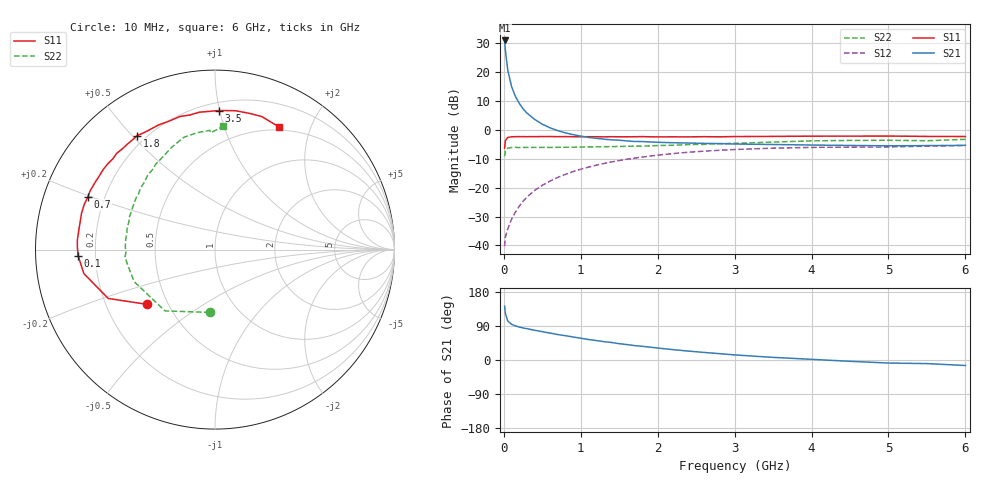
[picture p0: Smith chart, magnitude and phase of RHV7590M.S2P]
! SIEMENS Small Signal Semiconductors
! BFR106
! Si NPN RF Bipolar Junction Transistor in SOT23
! VCE = 0.75 V  IC = 90 mA
! Common Emitter S-Parameters:  August  1996
# GHz  S  MA  R  50
!  f  S11  S21  S12  S22
! GHz  MAG  ANG  MAG  ANG  MAG  ANG  MAG  ANG
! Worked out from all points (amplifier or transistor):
!   36 points, 10 MHz to 6 GHz, reference 50 ohm
!   highest |S21| = 31.0 dB at 10 MHz (marker M1)
!   |S21| within 3 dB of that: start of sweep to 19.03 MHz
!   unconditionally stable (mu >= 1): start of sweep to 13.64 MHz; 37.86 MHz to end of sweep
!   at 250 MHz: K = 1.56, MAG = 11.6 dB, |S12| = -24.7 dB
!   at 1.4 GHz: K = 1.28, MAG = 0.6 dB, |S12| = -11.1 dB
!   at 6 GHz: K = 1.04, MAG = -1.2 dB, |S12| = -5.4 dB
!   S11 on the Smith chart (normalised r, x): 10 MHz: 0.38, -0.31; 100 MHz: 0.13, -0.02; 700 MHz: 0.14, +0.20; 1.8 GHz: 0.17, +0.52; 3.5 GHz: 0.26, +1.00; 6 GHz: 0.46, +1.56
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0.01  0.4851 -141.0  35.68 141.9  0.0097 53.5  0.3513 -94.9
0.02  0.6541 -155.4  24.33 122.4  0.014 45.4  0.4407 -129.2
0.05  0.7425 -169.6  11.09 103.3  0.019 47.5  0.4847 -158.4
0.1  0.7635 -177.4  5.689 94.2  0.0284 58.0  0.4959 -171.1
0.15  0.7671 178.7  3.834 90.1  0.0376 64.0  0.5024 -175.6
0.2  0.7688 176.1  2.906 87.0  0.0478 67.7  0.4957 -178.6
0.25  0.7671 174.0  2.33 84.5  0.0584 69.1  0.4994 178.9
0.3  0.7665 172.1  1.968 82.7  0.0688 69.5  0.5001 177.4
0.4  0.7672 168.1  1.529 78.5  0.0895 69.9  0.5004 174.4
0.5  0.7705 164.8  1.261 74.8  0.1101 69.1  0.5003 171.7
0.6  0.7708 161.0  1.092 71.0  0.1303 67.9  0.499 169.6
0.7  0.7666 157.5  0.978 67.2  0.1505 66.5  0.5025 167.5
0.9  0.7661 151.3  0.831 60.7  0.1905 62.7  0.5037 162.7
1.1  0.7662 144.5  0.744 54.1  0.2275 59.0  0.5103 158.9
1.8  0.7689 124.3  0.632 36.1  0.34 44.4  0.5267 144.2
2.2  0.7624 114.5  0.602 27.3  0.3904 36.4  0.5444 136.1
2.6  0.767 104.6  0.587 20.0  0.4299 28.9  0.5644 128.4
3.5  0.7753 88.3  0.561 6.9  0.4849 14.2  0.6183 113.1
4.5  0.783 75.7  0.54 -3.5  0.5047 1.2  0.6591 98.6
5  0.7857 70.6  0.533 -8.0  0.5093 -3.8  0.6648 92.5
5.5  0.7749 65.9  0.537 -9.5  0.5244 -6.3  0.6516 92.0
6  0.7716 62.3  0.543 -14.5  0.5379 -12.1  0.6899 86.1
